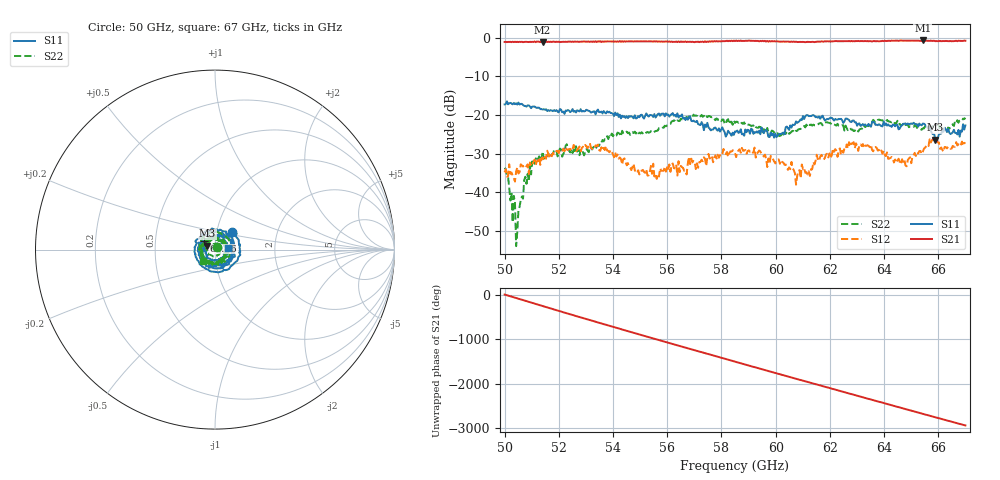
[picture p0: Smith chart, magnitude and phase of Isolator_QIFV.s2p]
!Agilent Technologies,E8361A,US42410132,A.06.03.05
!Agilent E8361A: A.06.03.05
!Date: Friday, July 11, 2008 14:59:50
!Correction: S11(Full 2 Port(1,2)) S21(Full 2 Port(1,2)) S12(Full 2 Port(1,2)) S22(Full 2 Port(1,2))
!S2P File: Measurements: S11, S21, S12, S22:
# Hz S  MA  R 50
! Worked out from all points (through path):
!   401 points, 50 GHz to 67 GHz, reference 50 ohm
!   highest |S21| = -0.76 dB at 65.43 GHz (marker M1); lowest = -1.2 dB at 51.4 GHz (marker M2)
!   group delay of S21, straight-line fit = 481 ps
!   lowest |S11| = -26.4 dB at 65.89 GHz (marker M3), VSWR 1.10, Z = 45.9 + j1.96 ohm
!   |S11| at or under -10 dB: start of sweep to end of sweep
!   |S22| runs from -54.0 to -19.9 dB; largest |S21 - S12| = 0.92
!   S11 on the Smith chart (normalised r, x): 50 GHz: 1.18, +0.24; 62.96 GHz: 0.88, +0.09; 67 GHz: 1.16, +0.02
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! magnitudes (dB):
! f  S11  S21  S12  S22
! 50 GHz  -17.3  -1.1  -34.9  -33.7
! 50.38 GHz  -17.2  -1.1  -37.3  -42.7
! 50.47 GHz  -17.3  -1.1  -33.6  -50.3
! 50.85 GHz  -17.5  -1.2  -32.8  -35.3
! 51.4 GHz  -18.6  -1.2  -31.0  -29.5
! 52.85 GHz  -19.1  -1.1  -28.6  -29.8
! 53.95 GHz  -19.6  -1.0  -29.5  -24.8
! 54.89 GHz  -20.8  -1.0  -35.1  -24.2
! 55.7 GHz  -19.6  -1.0  -36.0  -23.5
! 56.97 GHz  -21.5  -1.2  -31.9  -19.9
! 58.5 GHz  -24.3  -0.9  -30.0  -22.1
! 60.03 GHz  -25.8  -1.0  -31.8  -25.0
! 60.84 GHz  -21.9  -1.2  -34.5  -23.7
! 61.35 GHz  -20.2  -1.1  -34.1  -22.8
! 61.6 GHz  -20.4  -1.1  -31.9  -22.2
! 62.96 GHz  -21.9  -0.9  -27.4  -23.7
! 64.19 GHz  -22.8  -0.8  -31.3  -21.7
! 64.79 GHz  -22.2  -0.8  -33.1  -22.7
! 65.43 GHz  -22.3  -0.8  -29.6  -23.5
! 65.89 GHz  -26.4  -0.9  -25.9  -22.5
! 66.15 GHz  -24.1  -0.9  -29.1  -23.5
! 67 GHz  -22.7  -0.8  -27.4  -20.8
